PROGRAM PickAndPlaceTest
VAR
	//MoveAbs与Home的Action中所用到的绝对、相对定位相关功能块
    FB_MoveAbs                  : ARRAY[1..7] OF MC_MoveAbsolute;//前4个用于抓取时的绝对定位，后三个用于回零
	FB_MoveReL                  : MC_MoveRelative;               //用于C轴的相对定位（旋转）
	
	//X轴方向上的飞锯耦合、解耦、停止功能块
    fbGearInPosX		        : MC_GearInPos;
	fbGearOut					: MC_GearOut;
	FB_StopX                    : MC_Stop;
	
	//仿真测试时皮带相关功能块
    BeltAxis                    : Axis_ref;
    FB_SetBeltPosition          : MC_SetPosition;
	MC_MoveTestAxis             : MC_MoveVelocity;
	MC_TestAxisPower            : MC_Power;
	MC_BeltReset                : MC_Reset;
    
	//抓取过程中的触发位、标志位
	StartHome                   : BOOL;//开始回零
	IsHoming                    : BOOL;//是否正在回零
	PickPlace AT %Q*            : BOOL;//用于气阀的开合
	StartPickAndPlace           : BOOL;//开始抓取
	IsPickingOrPlacing          : BOOL;//是否正在抓取
	
	//模拟视觉程序发送的坐标所定义的结构体
	dmaterial                   : DUT_material;
	
	//Case步及其它功能块
	i                           : INT;//循环用变量
	MoveStep                    : INT;//抓取Case步
	HomingStep                  : INT;//回零Case步
	Ton1                        : TON;
	FB_Rising                   : R_Trig;//上升沿

	//NCI G代码功能块
	FB_BuildNciGroup            : CfgBuildExt3DGroup;//配置NCI通道
    FB_LoadNciProg              : ItpLoadProgEx;//加载G代码文件                 
	FB_StartGProg               : ItpStartStopEx;//启动停止
	FB_CfgReconfigGroup         : CfgReconfigGroup;//清除NCI通道
	FB_ItpResetGroup            : ItpResetEx2;//复位NCI通道
	L_Override                  : LREAL  :=100;  //通道速比
	ProgName                    : STRING(255):='Home.nc';//G代码文件名
	Gstep                       : INT;
    uiItpState                  : UDINT; //插补通道状态返回值
	StartGProHome               : BOOL; //G代码回零触发位
	
END_VAR

//调用飞锯相关功能块
FlayingSaw();
//调用绝对定位相关功能块
MoveAbs();
//调用回零程序（ST)
Home();
//调用回零程序（G代码）
GProgHome();


//轮询读取轴的状态
FOR i := 1 TO 7 BY 1 DO
    AxisArray[i].ReadStatus();
END_FOR
BeltAxis.ReadStatus();

//抓取逻辑
CASE MoveStep OF

0://初始化步，初始化各个触发位、标志位
  FOR i:=1 TO 4 DO 
	  FB_MoveAbs[i].Execute:=FALSE;
  END_FOR
  MC_TestAxisPower.Enable:=TRUE;
  FB_SetBeltPosition.Execute:=FALSE;
  MC_BeltReset.Execute:=FALSE;
  MC_MoveTestAxis.Execute:=FALSE;
  fbGearInPosX.Execute:=FALSE;
  fbGearOut.Execute:=FALSE;
  FB_StopX.Execute:=FALSE;
  IsPickingOrPlacing:=FALSE; 
  IF StartPickAndPlace=TRUE THEN //模拟仿真时，置位StartPickAndPlace变量则开始执行抓取动作，该变量与HMI界面的开始抓取按扭绑定
	 MoveStep:=10;	  
  END_IF  
  (*开始执行飞锯的标志位由视觉程序发出，当物料的最终坐标发送后，结构体中的bmaterial将会置位，此时，飞锯开始执行。
  IF dmaterial.bmaterial=TRUE THEN 
     StartPickAndPlace:=TRUE;
	 MoveStep:=10;	  
  END_IF*)

10://绝对定位到抓取点
  StartPickAndPlace:=FALSE; //开始抓取触发位复位
  IsPickingOrPlacing:=TRUE; //是否正在抓取标志位置位
  (*dmaterial.bmaterial:=FALSE; //实际执行时视觉的标志位复位*)
  MC_MoveTestAxis.Execute:=TRUE; //仿真时虚轴皮带使能
  FB_SetBeltPosition.Execute:=TRUE;//皮带当前位置置0，为飞锯耦合做准备
  FB_MoveAbs[1].Execute :=TRUE;//绝对定位机器人到Y轴坐标位置
  IF  FB_MoveAbs[1].Done THEN        //判断定位是否完成，若完成则跳到下一步
	  FB_MoveAbs[1].Execute:=FALSE;
	  FB_SetBeltPosition.Execute:=FALSE;
	  MoveStep:=20;
  END_IF
  IF  AxisArray[6].Status.Error THEN //判断定位是否有报错，若有则跳到999步，后续报错判断代码相同
	  FB_MoveAbs[1].Execute:=FALSE;
	  MoveStep:=999;
  END_IF
 
20://飞锯耦合
   fbGearInPosX.Execute:=TRUE;  //执行飞锯
   IF  fbGearInPosX.InSync THEN  //飞锯耦合标志位，若置True则代表机器人与皮带已经耦合，便可解耦开始进行抓取
	   fbGearInPosX.Execute:=FALSE;
	   MoveStep:=30;
   END_IF
   IF AxisArray[5].Status.Error THEN
	   fbGearInPosX.Execute:=FALSE;
	   MoveStep:=999;
   END_IF


30://飞锯解耦
  Ton1(IN:=TRUE, PT:=T#50MS , Q=> , ET=> );//跟随一段时间皮带后进行解耦
  IF Ton1.Q THEN
     fbGearOut.Execute:=TRUE;//触发解耦
     IF  fbGearOut.Done THEN
	     fbGearOut.Execute:=FALSE;
		 Ton1(IN:=FALSE, PT:=T#50MS , Q=> , ET=> );
         MoveStep:=40;
     END_IF
     IF  AxisArray[5].Status.Error THEN
	     fbGearOut.Execute:=FALSE;
         MoveStep:=999;
     END_IF
  END_IF
  
40:
  FB_MoveAbs[3].Execute:=TRUE;//Z轴下压进行抓取
  PickPlace:=1;//置位气阀，对物料进行吸取
  IF  FB_MoveAbs[3].Done THEN
	  FB_MoveAbs[3].Execute:=FALSE;
	  MoveStep:=50;
  END_IF
  IF  AxisArray[7].Status.Error THEN
	  FB_MoveAbs[3].Execute:=FALSE;
	  MoveStep:=999;
  END_IF
  
50:
  FB_MoveAbs[4].Execute:=TRUE;//Z轴抬升，回到抓取前的高度
  IF  FB_MoveAbs[4].Done THEN
	  FB_MoveAbs[4].Execute:=FALSE;
	  MoveStep:=60;
  END_IF
  IF  AxisArray[7].Status.Error THEN
	  FB_MoveAbs[4].Execute:=FALSE;
	  MoveStep:=999;
  END_IF

60:
  fb_Stopx.Execute:=TRUE;//抬升完成后便可停止X方向上的移动，使用stop功能块停止
  IF fb_Stopx.Done THEN
     fb_Stopx.Execute:=FALSE;
	 MoveStep:=70;
  END_IF 
  IF AxisArray[5].Status.Error THEN
	 fb_Stopx.Execute:=FALSE;
	 MoveStep:=999; 
  END_IF

70:
  FB_MoveAbs[2].Execute:=TRUE;//在Y轴方向上绝对定位，位移到旋切皮带的中点
  FB_MoveRel.Execute:=TRUE;//C轴相对定位对物料进行旋转
  IF  FB_MoveAbs[2].Done AND FB_MoveRel.Done  THEN
	  FB_MoveAbs[2].Execute:=FALSE;
	  FB_MoveRel.Execute:=FALSE;
	  MoveStep:=80;
  END_IF
  IF  AxisArray[6].Status.Error OR AxisArray[4].Status.Error THEN
	  FB_MoveAbs[2].Execute:=FALSE;
	  FB_MoveRel.Execute:=FALSE;
	  MoveStep:=999;
  END_IF
  
80:
  FB_MoveAbs[3].Execute:=TRUE;//Z轴再次下压准备松开气阀放下物料
  IF  FB_MoveAbs[3].Done THEN
	  FB_MoveAbs[3].Execute:=FALSE;
	  PickPlace:=0;
	  MoveStep:=90;
  END_IF
  IF  AxisArray[7].Status.Error THEN
	  FB_MoveAbs[3].Execute:=FALSE;
	  MoveStep:=999;
  END_IF
  
90:
   FB_MoveAbs[4].Execute:=TRUE;//放置完物料后讲Z轴抬升回原来的高度并返回初始步等待下一次的抓取信号
   IF  FB_MoveAbs[4].Done THEN
	   FB_MoveAbs[4].Execute:=FALSE;
	   MaterialNum:=MaterialNum+1;//此变量是为后续旋切所准备变量，代表物料数，当一个抓取循环结束后，该变量自加
	   MoveStep:=0;
   END_IF
   IF AxisArray[7].Status.Error THEN
	  FB_MoveAbs[4].Execute:=FALSE;
	  MoveStep:=999;
   END_IF

999://报错判断步
    fbGearOut.Execute:=TRUE;//解耦
	MaterialNum:=0;//清零物料数
	MC_BeltReset.Execute:=TRUE;//复位皮带
     IF  fbGearOut.Done AND MC_BeltReset.Done THEN //当解耦与皮带复位都完成后返回初始步
	     fbGearOut.Execute:=FALSE;
		 MC_BeltReset.Execute:=FALSE;
		 Ton1(IN:=FALSE, PT:=T#100MS , Q=> , ET=> );
         MoveStep:=0;
     END_IF
      
 END_CASE

ACTION FlayingSaw:
//该Action用于定义飞锯耦合时所用到的一些功能块

//皮带当前位置设0
FB_SetBeltPosition(
	Axis:=BeltAxis , 
	Execute:= , 
	Position:=0 , 
 );
 

//飞锯耦合功能块
fbGearInPosX(
	Master:=BeltAxis ,//主轴为皮带 
	Slave:=AxisArray[5] , //从轴为机器人的X方向
	Execute:= , 
	RatioNumerator:=1 , //齿轮比设定为1：1
	RatioDenominator:=1 , 
	MasterSyncPosition:=466,//主轴耦合点采用9点标定中两个坐标系的偏移值来模拟抓取点 
	SlaveSyncPosition:=0,//机器人X轴耦合点就采用X轴的零点位置来进行模拟
	SyncMode:= , 
	MasterStartDistance:= , 
	Velocity:= , 
	Acceleration:=, 
	Deceleration:= , 
	Jerk:= , 
);


//飞锯解耦功能块
fbGearOut(
	Slave:=AxisArray[5] , 
  );
 

//X轴方向停止
FB_StopX(
	Axis:=AxisArray[5] , 
	Execute:= , 
);


//移动皮带
MC_MoveTestAxis(
	Axis:=BeltAxis , 
	Execute:=  , 
	Velocity:=70, 
 );

//使能皮带 
MC_TestAxisPower(
	Axis:=Beltaxis , 
	Enable:= , 
	Enable_Positive:=1 , 
	Enable_Negative:=1 , 
 );

//皮带复位
MC_BeltReset(
	Axis:=BeltAxis , 
	Execute:= , 
	 );
END_ACTION

ACTION GProgHome:
(*NCI通道状态，通常用作标志位,uiItpState返回值代表着当前插补通道的状态，其中几个重要的状态：
  1：ITP_STATE_IDLE     该状态未加载任何G代码程序或是刚执行完复位功能，插补通道处于空闲状态。若当前执行G代码停止也会进入该状态。
  2: ITP_STATE_READY    成功导入G代码程序，插补通道进入准备状态。当G代码程序被完整执行完，插补通道也会进入该状态
  5: ITP_STATE_RUNNING  正在运行G代码
 12: ITP_STATE_ABORTED  如果在G代码运行过程中出现报错，插补通道立即进入该模式，当前报错代码也会出现在通道状态中*)
uiItpState	:=	ItpGetStateInterpreter( stKinToPlc);
(*设置NCI通道的override*)
ItpSetOverridePercent(fOverridePercent:=L_Override, sPlcToNci:=stPlcToKin);

//配置插补通道功能块，设定XYZ插补轴
FB_BuildNciGroup(
	bExecute:= , 
	nGroupId:=13 , 
	nXAxisId:=AxisArray[5].NcToPlc.AxisId , 
	nYAxisId:=AxisArray[6].NcToPlc.AxisId , 
	nZAxisId:=AxisArray[7].NcToPlc.AxisId, 
	nQ1AxisId:=0 , 
	nQ2AxisId:=0 , 
	nQ3AxisId:=0 , 
	nQ4AxisId:=0 , 
	nQ5AxisId:=0, 
	tTimeOut:=T#300MS ,  );

//上载G代码功能块 
FB_LoadNciProg(
	sNciToPlc:=stKinToPlc , 
	bExecute:= , 
	sPrg:=ProgName , 
	nLength:=INT_TO_UDINT(Len(ProgName)), 
	tTimeOut:=T#300MS , );

//运行G代码功能块	
FB_StartGProg(
	bStart:= , 
	bStop:= , 
	tTimeOut:= , 
	sNciToPlc:=stKinToPlc , 
	bBusy=> , 
	bErr=> , 
	nErrId=> );

//清除插补通道功能块	
FB_CfgReconfigGroup(
	bExecute:= , 
	nGroupId:=13 , 
	tTimeOut:=T#300MS , );

//复位插补通道功能块	
FB_ItpResetGroup(
	bExecute:= , 
	tTimeOut:=T#300MS , 
	sNciToPlc:=stKinToPlc ,  );
	
CASE Gstep OF
0://初始化步，复位标志位及触发位
  FB_BuildNciGroup.bExecute:=FALSE;
  FB_LoadNciProg.bExecute:=FALSE;
  FB_CfgReconfigGroup.bExecute:=FALSE;
  FB_StartGProg.bStart:=FALSE;
  FB_StartGProg.bStop:=FALSE;
  IsHoming:=FALSE;//是否正在回零标志位
  //Gstep:=10; 
  IF StartGProHome=TRUE THEN
	 Gstep:=10; 
  END_IF

10: 
  FB_BuildNciGroup.bExecute:=TRUE;
  IsHoming:=TRUE; //正在回零
  IF uiItpState=1 OR uiItpState= 2 THEN//判断NCI通道状态，初次执行时返回值为1，后续执行返回值为2
 	 Gstep:=20;
  END_IF
  IF FB_BuildNciGroup.bErr OR uiItpState= 12 THEN//报错判断步功能块报错或插补通道报错,后续报错判断步都为如此
	 Gstep:=99;
  END_IF
  
20: 
  FB_LoadNciProg.bExecute:=TRUE;
  IF  uiItpState=2 THEN  //上载G代码文件后NCI通道状态为2 
	  Gstep:=30;
  END_IF
  IF FB_LoadNciProg.bErr OR uiItpState= 12 THEN 
	 Gstep:=99;
  END_IF
 
30:
  FB_StartGProg.bStart:=TRUE; //运行G代码文件进行回零
  IF uiItpState=5 THEN  //正在运行时NCI通道状态为5
     Gstep:=40;
  END_IF
  IF FB_StartGProg.bErr OR uiItpState= 12 THEN 
	 Gstep:=99;
  END_IF

40:
  IF NOT FB_StartGProg.bBusy AND  uiItpState=2 THEN //等待是否执行完成
     StartGProHome:=FALSE;
	 FB_CfgReconfigGroup.bExecute:=TRUE; //执行完成后必须清楚NCI通道，否则与抓取程序的配置冲突
	 Gstep:=0;
  END_IF
  IF FB_CfgReconfigGroup.bErr OR uiItpState= 12 THEN 
	 Gstep:=99;
  END_IF
  
99://报错处理步,复位NCI通道并返回初始步 
  StartGProHome:=FALSE;
  FB_ItpResetGroup.bExecute:=TRUE;
  IF NOT FB_ItpResetGroup.bBusy THEN
	 Gstep:=0; 
  END_IF
END_CASE
END_ACTION

ACTION Home:
//TC2_MC2库的机器人回零功能，用绝对定位进行回零

//X轴绝对定位
FB_MoveAbs[5](
	Axis:=AxisArray[5] , 
	Execute:= , 
	Position:=0, 
	Velocity:=300 ,
    Acceleration:=15000,
	Deceleration:=15000 , 
	Jerk:=30000 ,
 );

//Y轴绝对定位 
FB_MoveAbs[6](
	Axis:=AxisArray[6] , 
	Execute:= , 
	Position:=0, 
	Velocity:=300 ,
    Acceleration:=15000,
	Deceleration:=15000 , 
	Jerk:=30000 ,
 );
 
//Z轴绝对定位 
FB_MoveAbs[7](
	Axis:=AxisArray[7] , 
	Execute:= , 
	Position:=30, 
	Velocity:=80 ,
    Acceleration:=15000,
	Deceleration:=15000 , 
	Jerk:=30000 
 );
 
CASE HomingStep OF 
0://初始化步
   FB_MoveAbs[5].Execute:=FALSE;
   FB_MoveAbs[6].Execute:=FALSE;
   FB_MoveAbs[7].Execute:=FALSE;
   IsHoming:=FALSE;//是否正在回零标志位
   IF StartHome=TRUE THEN //回零功能触发位
	  HomingStep:=10;
   END_IF
   
10://x轴回零位
   IsHoming:=TRUE;//正在回零
   StartHome:=FALSE;
   FB_MoveAbs[5].Execute:=TRUE;
   IF FB_MoveAbs[5].Done THEN
	  FB_MoveAbs[5].Execute:=FALSE;
	  HomingStep:=20;
   END_IF
   IF FB_MoveAbs[5].Error THEN//报错判断步
	  FB_MoveAbs[5].Execute:=FALSE;
	  HomingStep:=0;
   END_IF

20: //Y轴回零位
   FB_MoveAbs[6].Execute:=TRUE;
   IF FB_MoveAbs[6].Done THEN
	  FB_MoveAbs[6].Execute:=FALSE;
	  HomingStep:=30;
   END_IF
   IF FB_MoveAbs[6].Error THEN
	  FB_MoveAbs[6].Execute:=FALSE;
	  HomingStep:=0;
   END_IF

30://Z轴返回初始位置
   FB_MoveAbs[7].Execute:=TRUE;
   IF FB_MoveAbs[7].Done THEN
	  FB_MoveAbs[7].Execute:=FALSE;
	  HomingStep:=0;
   END_IF
   IF FB_MoveAbs[7].Error THEN
	  FB_MoveAbs[7].Execute:=FALSE;
	  HomingStep:=0;
   END_IF
   
END_CASE
END_ACTION

ACTION MoveAbs:
//该Action用于定义机器人抓取过程中的绝对定位与相对定位功能块

//绝对定位到Y轴的抓取点
FB_MoveAbs[1](
	Axis:=AxisArray[6] , 
	Execute:= , 
	Position:= dmaterial.lrCenterY, //该引脚在配合视觉时需要填写视觉程序发送的Y坐标,此处填写模拟结构体中的Y轴数值
	Velocity:=300 ,
    Acceleration:=15000,
	Deceleration:=15000 , 
	Jerk:=30000 , 
 );  

//Y轴绝对定位到旋切皮带的中点
FB_MoveAbs[2](
	Axis:=AxisArray[6] , 
	Execute:= , 
	Position:=85, 
	Velocity:=300 ,
    Acceleration:=15000,
	Deceleration:=15000 , 
	Jerk:=30000 , 
 );
 
//Z轴下压进行抓取
FB_MoveAbs[3](
	Axis:=AxisArray[7] , 
	Execute:= , 
	Position:=15, 
	Velocity:=150 ,
    Acceleration:=15000,
	Deceleration:=15000 , 
	Jerk:=30000 , 
 );

//Z轴上升 
FB_MoveAbs[4](
	Axis:=AxisArray[7] , 
	Execute:= , 
	Position:=30, 
	Velocity:=150 ,
    Acceleration:=15000,
	Deceleration:=15000 , 
	Jerk:=30000 , 
 );

//C相对定位轴相对定位进行物料的旋转 
FB_MoveReL(
	Axis:=AxisArray[4] , 
	Execute:= , 
	Distance:=dmaterial.lrAngle , //该引脚在配合视觉时需要填写视觉程序发送的Angle值,此处填写结构体中的Angle值
	Velocity:=150 ,
    Acceleration:=15000,
	Deceleration:=15000 , 
	Jerk:=30000 , 
 );
END_ACTION

END_PROGRAM
